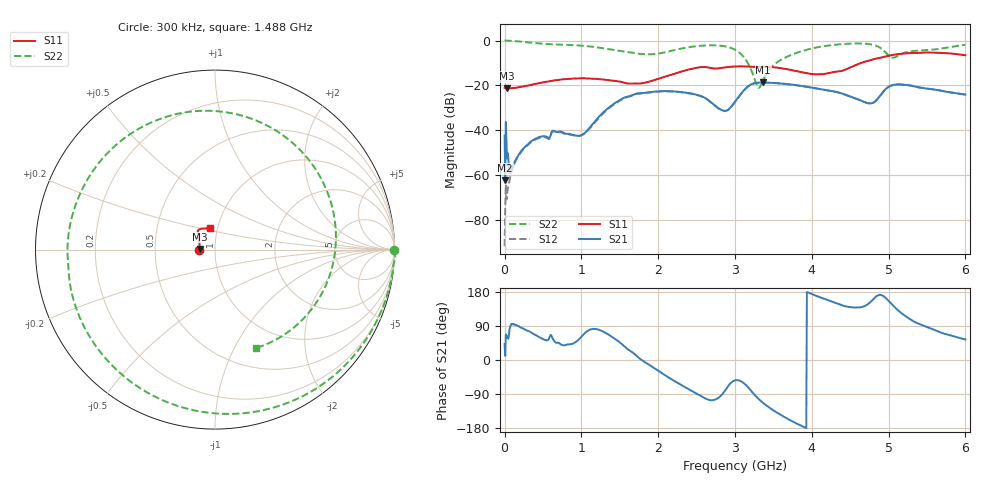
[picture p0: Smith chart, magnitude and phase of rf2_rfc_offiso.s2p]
!Agilent Technologies,M9375A,MY55441453,A.02.50.04
!Agilent M9375A: A.02.50.04
!Date: Monday, December 12, 2016 11:27:08
!Correction: S11(Full 2 Port(1,2))
!S21(Full 2 Port(1,2))
!S12(Full 2 Port(1,2))
!S22(Full 2 Port(1,2))
!S2P File: Measurements: S11, S21, S12, S22:
# Hz S  dB  R 50
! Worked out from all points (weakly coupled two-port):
!   751 points, 300 kHz to 6 GHz, reference 50 ohm
!   highest |S21| = -18.74 dB at 3.368 GHz (marker M1); lowest = -62.5 dB at 8.3 MHz (marker M2)
!   lowest |S11| = -21.4 dB at 32.3 MHz (marker M3), VSWR 1.19, Z = 42.1 + j0.249 ohm
!   |S11| at or under -10 dB: start of sweep to 4.643 GHz
!   |S22| runs from -21.1 to 0.0 dB; largest |S21 - S12| = 0.015
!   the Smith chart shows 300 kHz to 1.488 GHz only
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300000  -21.07 -177.1  -42.47 41.6  -91.92 32.7  -0.03 -0.2
8299600  -21.17 179.8  -62.52 10.8  -74.66 97.4  0.05 -2.4
3.22984e7  -21.37 178.0  -52.73 63.0  -68.57 93.0  -0.04 -9.7
8.0296e7  -21.32 172.4  -58.96 91.5  -59.83 102.2  -0.13 -23.7
2.80286e8  -20.27 154.7  -47.05 79.1  -47.35 78.8  -0.70 -82.6
5.60272e8  -18.32 140.6  -43.22 52.2  -43.78 52.8  -1.57 -162.6
1.00025e9  -16.87 129.6  -42.29 61.3  -42.40 60.8  -2.27 87.6
1.264237e9  -17.35 119.9  -32.79 76.9  -33.24 77.0  -3.34 8.6
1.520224e9  -18.47 99.8  -26.18 43.1  -26.46 44.4  -4.70 -78.3
1.768212e9  -19.18 75.1  -23.54 2.3  -23.70 3.5  -5.95 -159.5
2.0002e9  -17.13 53.8  -22.71 -28.4  -22.80 -27.5  -5.83 123.4
2.560172e9  -11.86 29.6  -24.85 -95.4  -24.94 -95.1  -2.31 8.1
3.00015e9  -11.58 37.9  -27.39 -53.7  -27.49 -53.5  -4.08 -69.8
3.176141e9  -11.66 40.2  -20.31 -73.1  -20.40 -72.7  -10.65 -127.8
3.296135e9  -11.68 43.2  -18.83 -100.7  -18.89 -100.1  -20.80 140.6
3.368132e9  -11.66 43.7  -18.74 -113.6  -18.79 -113.1  -17.59 55.1
3.624119e9  -12.49 39.3  -19.26 -148.1  -19.28 -147.7  -8.14 -36.6
4.0001e9  -14.98 10.7  -21.03 174.1  -21.06 174.3  -3.53 -102.8
4.688066e9  -9.49 -49.7  -27.50 142.3  -27.54 142.6  -1.40 -153.6
5.00005e9  -6.80 -51.4  -20.70 156.3  -20.74 156.5  -6.66 -175.2
5.240038e9  -5.68 -51.7  -19.89 113.0  -19.90 113.1  -5.15 -161.9
6e9  -6.56 -43.1  -24.16 54.1  -24.18 54.2  -1.84 98.9
